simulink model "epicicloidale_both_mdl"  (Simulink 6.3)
settings: Solver=ode45  StartTime=0.0  StopTime=10.0  RelTol=1e-3
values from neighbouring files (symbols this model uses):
  b_c = kb*J_c    (= 4.94590955184)    [architetture_epicicloidale.m]    (also in architetture_epicicloidale_cont.m; architetture_epicicloidale_HEV.m = 92.8974810391; architetture_epicicloidale_prova.m; architetture_HEV_controllo.m = 9.28974810391)
  b_r = kb*J_r    (= 218.026030555)    [architetture_epicicloidale.m]    (also in architetture_epicicloidale_cont.m; architetture_epicicloidale_HEV.m; architetture_epicicloidale_prova.m; architetture_HEV_controllo.m = 21.8026030555)
  b_s = kb*J_s    (= 8.12277148259)    [architetture_epicicloidale.m]    (also in architetture_epicicloidale_cont.m; architetture_epicicloidale_HEV.m = 4.94590955184; architetture_epicicloidale_prova.m; architetture_HEV_controllo.m = 0.494590955184)
  b_sc = kb*J_sc    (= 92.8974810391)    [architetture_epicicloidale.m]    (also in architetture_epicicloidale_cont.m; architetture_epicicloidale_prova.m; epicicloidale.m; epicicloidale_da_solo.m)
  d_cs = d0    (= 10)    [architetture_epicicloidale.m]    (also in architetture_epicicloidale_cont.m; architetture_epicicloidale_prova.m; epicicloidale.m; epicicloidale_da_solo.m)
  d_sr = d0    (= 10)    [architetture_epicicloidale.m]    (also in architetture_epicicloidale_cont.m; architetture_epicicloidale_prova.m; epicicloidale.m; epicicloidale_da_solo.m)
  J_c = 1.3*0.5*pi*rho_acc*hc*r_c^4    (= 0.0494590955184)    [architetture_epicicloidale.m]    (also in architetture_epicicloidale_cont.m; architetture_epicicloidale_HEV.m = 0.928974810391; architetture_epicicloidale_prova.m; architetture_HEV_controllo.m = 0.928974810391)
  J_r = 0.5*pi*rho_acc*(hr*r_ri^4 + h_ring*(r_re^4-r_ri^4))    (= 2.18026030555)    [architetture_epicicloidale.m]    (also in architetture_epicicloidale_cont.m; architetture_epicicloidale_HEV.m; architetture_epicicloidale_prova.m; architetture_HEV_controllo.m)
  J_s = Nr_sat*0.5*pi*rho_acc*(hs*r_s^4 + hc*r_s^4)    (= 0.0812277148259)    [architetture_epicicloidale.m]    (also in architetture_epicicloidale_cont.m; architetture_epicicloidale_HEV.m = 0.0494590955184; architetture_epicicloidale_prova.m; architetture_HEV_controllo.m = 0.0494590955184)
  J_sc = Nr_sat*(r_c+r_s)^2*rho_acc*pi*(hs*r_s^2 + hc*r_s^2)    (= 0.928974810391)    [architetture_epicicloidale.m]    (also in architetture_epicicloidale_cont.m; architetture_epicicloidale_prova.m; epicicloidale.m; epicicloidale_da_solo.m)
  K_cs = K0    (= 10000000)    [architetture_epicicloidale.m]    (also in architetture_epicicloidale_cont.m; architetture_epicicloidale_prova.m; epicicloidale.m; epicicloidale_da_solo.m)
  K_sr = K0    (= 10000000)    [architetture_epicicloidale.m]    (also in architetture_epicicloidale_cont.m; architetture_epicicloidale_prova.m; epicicloidale.m; epicicloidale_da_solo.m)
  Nr_sat = 4    [architetture_epicicloidale.m]    (also in architetture_epicicloidale_cont.m; architetture_epicicloidale_HEV.m; architetture_epicicloidale_prova.m; architetture_HEV_controllo.m)
  r_c = r_ri-2*r_s    (= 0.101859163579)    [architetture_epicicloidale.m]    (also in architetture_epicicloidale_cont.m; architetture_epicicloidale_prova.m; epicicloidale.m; epicicloidale_da_solo.m)
  r_ri = xds*Nr/(2*pi)    (= 0.248281711223)    [architetture_epicicloidale.m]    (also in architetture_epicicloidale_cont.m; architetture_epicicloidale_prova.m; epicicloidale.m; epicicloidale_da_solo.m)
  r_s = xds*Ns/(2*pi)    (= 0.0732112738223)    [architetture_epicicloidale.m]    (also in architetture_epicicloidale_cont.m; architetture_epicicloidale_HEV.m = 0.101859163579; architetture_epicicloidale_prova.m; architetture_HEV_controllo.m = 0.101859163579)
  Tau_c = 0*N*metri    (= 0)    [architetture_epicicloidale.m]    (also in architetture_epicicloidale_cont.m; architetture_epicicloidale_prova.m; epicicloidale.m; epicicloidale_confronto_statico_elastico.m = 10)
  Tau_r = 0*N*metri    (= 0)    [architetture_epicicloidale.m]    (also in architetture_epicicloidale_cont.m; architetture_epicicloidale_prova.m; epicicloidale.m; epicicloidale_confronto_statico_elastico.m = 20)
  Tau_sc = 200*N*metri    (= 200)    [architetture_epicicloidale.m]    (also in architetture_epicicloidale_cont.m = 50; architetture_epicicloidale_prova.m = 50; epicicloidale.m = 4; epicicloidale_da_solo.m = 4)
  Tc = 0.05*ms    (= 5e-05)    [architetture_epicicloidale.m]    (also in architetture_epicicloidale_cont.m; architetture_epicicloidale_HEV.m; architetture_epicicloidale_prova.m; architetture_HEV_controllo.m)
  Wc_0 = 0*0.1*rad/secondo    (= 0)    [architetture_epicicloidale.m]    (also in architetture_epicicloidale_cont.m; architetture_epicicloidale_HEV.m; architetture_epicicloidale_prova.m; Confronto_CVT_EMR.m)
  Wr_0 = Sys1.C(3,:)*[Wc_0; Wsc_0]    [architetture_epicicloidale.m]    (also in Confronto_CVT_EMR.m = 0; epicicloidale.m; epicicloidale_confronto_statico_elastico.m = [-r_s/r_r, 1+r_s/r_r]*[Ws_0; Wc_0]; epicicloidale_da_solo.m = [ -1/r_ri*r_c, (r_c+r_ri)/r_ri]*[Wc_0; Wsc_0])
  Wsc_0 = -0*0.2*rad/secondo    (= 0)    [architetture_epicicloidale.m]    (also in architetture_epicicloidale_cont.m; architetture_epicicloidale_HEV.m; architetture_epicicloidale_prova.m; epicicloidale.m = -0.2)

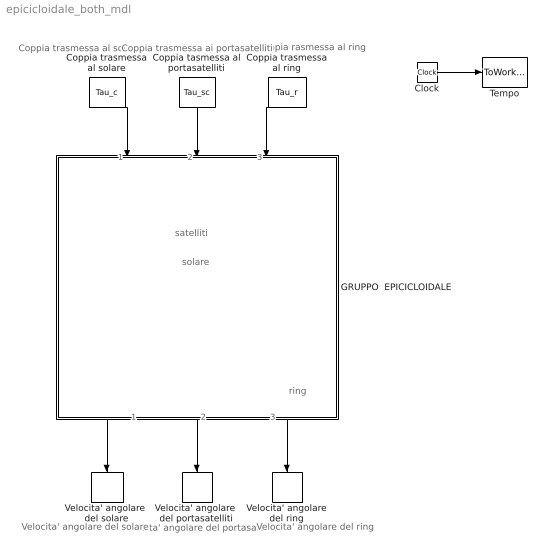
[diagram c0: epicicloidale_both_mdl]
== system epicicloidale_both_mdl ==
  note: solare
  note: satelliti
  note: ring
  note: Velocita' angolare del portasatelliti
  note: Velocita' angolare del ring
  note: Velocita' angolare del solare
  note: Coppia rasmessa al ring
  note: Coppia trasmessa al solare
  note: Coppia trasmessa ai portasatelliti
  Clock : Clock
  Coppia tasmessa al portasatelliti : Constant  Orientation=down  Value=Tau_sc
  Coppia trasmessa al ring : Constant  Orientation=down  Value=Tau_r
  Coppia trasmessa al solare : Constant  Orientation=down  Value=Tau_c
  GRUPPO  EPICICLOIDALE : Subsystem  Orientation=down  mask(POG Gruppo epicicloidale){Par_solare=[J_c, b_c, r_c], Par_satelliti=[J_s, J_sc, b_s, b_sc, r_s, Nr_sat], Par_ring=[J_r, b_r, r_ri], Tipo_di_Modello=Modello ridotto Wc-Wsc, Cond_in_Wc_Wsc=[Wc_0,  Wsc_0], Cond_in_Wsc_Wr=[Wsc_0,  Wr_0], Cond_in_Wc_Wr=[Wc_0,  Wr_0], Solare_Satelliti=[K_cs, d_cs], Satelliti_Ring=[K_sr, d_sr], Cond_in=[Wc_0, Wsc_0,Wr_0]}
      mask prompts: Par_solare "Parametri Solare: [J_c, b_c, r_c]-->[kg*m^2,N*m*s/rad,m]"; Par_satelliti "Parametri Satelliti: [J_s, J_sc, b_s, b_sc, r_s, Nr_sat]-->[kg*m^2,N*m*s/rad,m]"; Par_ring "Parametri Ring: [J_r, b_r, r_ri]-->[kg*m^2,N*m*s/rad,m,m]"; Tipo_di_Modello "Tipo di modello"; Cond_in_Wc_Wsc "Condizioni iniziali: [Wc_0,  Wsc_0]-->[rad/s]"; Cond_in_Wsc_Wr "Condizioni iniziali: [Wsc_0,  Wr_0]-->[rad/s]"; Cond_in_Wc_Wr "Condizioni iniziali: [Wc_0,  Wr_0]-->[rad/s]"; Solare_Satelliti "Solare-Satelliti: [K_cs, d_cs]-->[N/m,N*m*s/rad]"; Satelliti_Ring "Satelliti-Ring: [K_sr, d_sr]-->[N/m,N*m*s/rad]"; Cond_in "Condizioni iniziali: [Wc_0,  Wsc_0, Wr_0]-->[rad/s]"
      mask help: Gruppo epicicloidale: [J_c, J_s, J_r, J_sc]= Inerzie di: solare, satelliti, ring, solare-ssatelliti; [b_c, b_s, b_r]= Attriti di: solare, satelliti, ring; [r_c, r_s, r_ri, r_re]= Raggi di: solare, satelliti, ring(interno ed esterno); [Nr_sat]= Numero Satelliti; [K_cs, K_sr]= Elasticita' tra solare-satelliti e tra satelliti-ring; [b_sc]= Attriti tra solare-satelliti; [d_cs, d_sr]= Elementi della matrice D; [Wc_0, Wsc_0, Wr_0]=Velocita' iniziali di solare, satelliti, portasatelliti, ring;
      mask init:
      | J_c=double(Par_solare(1));          
      | b_c=double(Par_solare(2));            
      | r_c=double(Par_solare(3));           
      | %
      | J_s=double(Par_satelliti(1));            
      | J_sc=double(Par_satelliti(2));            
      | b_s=double(Par_satelliti(3));            
      | b_sc=double(Par_satelliti(4));            
      | r_s=double(Par_satelliti(5));            
      | Nr_sat=double(Par_satelliti(6));           
      | %
      | J_r=double(Par_ring(1));             
      | b_r=double(Par_ring(2));            
      | r_ri=double(Par_ring(3));                  
      | %
      | %%%%%%%%%%%%%%%%%%%%%%%%%%%%%%%%%%%%%%%%%%%%%%%%%%%%%%%%%%%%%%%%%%%%%%%%%%%
      | %   Modello esteso e modelli ridotti
      | %%%%%%%%%%%%%%%%%%%%%%%%%%%%%%%%%%%%%%%%%%%%%%%%%%%%%%%%%%%%%%%%%%%%%%%%%%%
      | if Tipo_di_Modello=='Modello esteso        '
      |     %
      |     K_cs=double(Solare_Satelliti(1));
      |     d_cs=double(Solare_Satelliti(2));
      |     if(K_cs==0)
      |         K_cs=inf;
      |     end
      |     %
      |     K_sr=double(Satelliti_Ring(1));
      |     d_sr=double(Satelliti_Ring(2));
      |     if(K_sr==0)
      |         K_sr=inf;
      |     end
      |     %
      |     %
      |     L=[ J_c,      0,      0,      0,      0,      0;
      |           0, 1/K_cs,      0,      0,      0,      0;
      |           0,      0,    J_s,      0,      0,      0;
      |           0,      0,      0,   J_sc,      0,      0;
      |           0,      0,      0,      0, 1/K_sr,      0;
      |           0,      0,      0,      0,      0,    J_r];
      |     %
      |     A=- [-b_c-r_c^2*d_cs,    -r_c,                -r_c*d_cs*r_s,                   r_c^2*d_cs,      0,                  0;
      |         r_c,                    0,                          r_s,                         -r_c,      0,                  0;
      |         -r_c*d_cs*r_s,       -r_s,   -b_s-d_cs*r_s^2-d_sr*r_s^2,   r_c*d_cs*r_s-d_sr*r_s*r_ri,   -r_s,      d_sr*r_s*r_ri;
      |         r_c^2*d_cs,           r_c,   r_c*d_cs*r_s-d_sr*r_s*r_ri, -b_sc-r_c^2*d_cs-d_sr*r_ri^2,  -r_ri,        d_sr*r_ri^2;
      |         0,                      0,                          r_s,                         r_ri,      0,              -r_ri;
      |         0,                      0,                d_sr*r_s*r_ri,                  d_sr*r_ri^2,   r_ri,   -b_r-d_sr*r_ri^2];
      |     %
      |     B=[ 1, 0, 0;
      |         0, 0, 0;
      |         0, 0, 0;
      |         0, 1, 0;
      |         0, 0, 0;
      |         0, 0, 1];
      |     %
      |     C=[ 1, 0, 0, 0, 0, 0;
      |         0, 0, 0, 1, 0, 0;
      |         0, 0, 0, 0, 0, 1];
      |     %
      |     Wc_0=double(Cond_in(1));
      |     Wsc_0=double(Cond_in(2));
      |     Wr_0=double(Cond_in(3));
      |     Ws_0=r_c*(Wsc_0-Wc_0)/r_s;
      |     Ws_sc_0=[Ws_0 Wsc_0];
      |     %
      |     We_0=[Wc_0 0 Ws_sc_0 0 Wr_0 ];
      |     %
      | elseif Tipo_di_Modello=='Modello ridotto Wc-Wsc'
      |     L = [ (J_c*r_s^2*r_ri^2+r_ri^2*r_c^2*J_s+J_r*r_s^2*r_c^2)/r_s^2/r_ri^2,                                        -r_c*(r_ri^2*r_c*J_s+J_r*r_s^2*r_c+J_r*r_s^2*r_ri)/r_s^2/r_ri^2;
      |           -r_c*(r_ri^2*r_c*J_s+J_r*r_s^2*r_c+J_r*r_s^2*r_ri)/r_s^2/r_ri^2, (J_r*r_s^2*r_c^2+2*J_r*r_s^2*r_ri*r_c+J_r*r_s^2*r_ri^2+r_ri^2*r_c^2*J_s+r_ri^2*J_sc*r_s^2)/r_s^2/r_ri^2];
      |     %
      |     A=-[ -(b_c*r_s^2*r_ri^2+r_c^2*r_ri^2*b_s+b_r*r_s^2*r_c^2)/r_s^2/r_ri^2,                                          r_c*(r_c*r_ri^2*b_s+b_r*r_s^2*r_c+b_r*r_s^2*r_ri)/r_s^2/r_ri^2;
      |         r_c*(r_c*r_ri^2*b_s+b_r*r_s^2*r_c+b_r*r_s^2*r_ri)/r_s^2/r_ri^2,    -(b_sc*r_s^2*r_ri^2+r_c^2*r_ri^2*b_s+b_r*r_s^2*r_c^2+2*b_r*r_s^2*r_c*r_ri+b_r*r_s^2*r_ri^2)/r_s^2/r_ri^2];
      |     %
      |     B= [  1,    0,     -1/r_ri*r_c;
      |           0,    1, (r_c+r_ri)/r_ri];
      |     %
      |     C= [            1,               0;
      |                     0,               1;
      |           -1/r_ri*r_c, (r_c+r_ri)/r_ri];
      |     %
      |     Wc_0=double(Cond_in_Wc_Wsc(1));
      |     Wsc_0=double(Cond_in_Wc_Wsc(2));
      |     We_0=[Wc_0 Wsc_0];
      |     %
      | elseif Tipo_di_Modello=='Modello ridotto Wsc-Wr'
      |     L= [ (J_sc*r_c^2*r_s^2+J_c*r_s^2*r_c^2+2*J_c*r_s^2*r_c*r_ri+J_c*r_s^2*r_ri^2+r_ri^2*J_s*r_c^2)/r_c^2/r_s^2,   -r_ri*(J_c*r_s^2*r_c+J_c*r_s^2*r_ri+r_ri*J_s*r_c^2)/r_c^2/r_s^2;
      |          -r_ri*(J_c*r_s^2*r_c+J_c*r_s^2*r_ri+r_ri*J_s*r_c^2)/r_c^2/r_s^2,                                        (J_r*r_c^2*r_s^2+J_c*r_s^2*r_ri^2+r_ri^2*J_s*r_c^2)/r_c^2/r_s^2];
      | 
      |     A=-[ -(b_sc*r_c^2*r_s^2+b_c*r_s^2*r_c^2+2*b_c*r_s^2*r_c*r_ri+b_c*r_s^2*r_ri^2+r_ri^2*b_s*r_c^2)/r_c^2/r_s^2,     r_ri*(b_c*r_s^2*r_c+b_c*r_s^2*r_ri+r_ri*b_s*r_c^2)/r_c^2/r_s^2;
      |          r_ri*(b_c*r_s^2*r_c+b_c*r_s^2*r_ri+r_ri*b_s*r_c^2)/r_c^2/r_s^2,                                          -(b_r*r_c^2*r_s^2+b_c*r_s^2*r_ri^2+r_ri^2*b_s*r_c^2)/r_c^2/r_s^2];
      | 
      |     B= [ (r_c+r_ri)/r_c,    1,   0;
      |             -1/r_c*r_ri,    0,   1];
      | 
      |     C= [ (r_c+r_ri)/r_c,  -1/r_c*r_ri;
      |                       1,            0;
      |                       0,            1];
      |     %
      |     Wsc_0=double(Cond_in_Wsc_Wr(1));
      |     Wr_0=double(Cond_in_Wsc_Wr(2));
      |     We_0=[Wsc_0 Wr_0];
      |     %
      | elseif Tipo_di_Modello=='Modello ridotto  Wc-Wr'
      |     L= [ (J_c*r_s^2*r_c^2+2*J_c*r_s^2*r_c*r_ri+J_c*r_s^2*r_ri^2+r_ri^2*r_c^2*J_s+r_c^2*J_sc*r_s^2)/r_s^2/(r_c+r_ri)^2,                                                        r_c*r_ri*(-r_ri*r_c*J_s+J_sc*r_s^2)/r_s^2/(r_c+r_ri)^2;
      |           r_c*r_ri*(-r_ri*r_c*J_s+J_sc*r_s^2)/r_s^2/(r_c+r_ri)^2,                                                      (J_r*r_s^2*r_c^2+2*J_r*r_s^2*r_c*r_ri+J_r*r_s^2*r_ri^2+r_ri^2*r_c^2*J_s+r_ri^2*J_sc*r_s^2)/r_s^2/(r_c+r_ri)^2];
      | 
      |     A=-[-(b_c*r_s^2*r_c^2+2*b_c*r_s^2*r_c*r_ri+b_c*r_s^2*r_ri^2+r_c^2*r_ri^2*b_s+r_c^2*r_s^2*b_sc)/r_s^2/(r_c+r_ri)^2,                                                        -r_c*r_ri*(-r_c*r_ri*b_s+r_s^2*b_sc)/r_s^2/(r_c+r_ri)^2;
      |         -r_c*r_ri*(-r_c*r_ri*b_s+r_s^2*b_sc)/r_s^2/(r_c+r_ri)^2,                                                       -(b_r*r_s^2*r_c^2+2*b_r*r_s^2*r_c*r_ri+b_r*r_s^2*r_ri^2+r_c^2*r_ri^2*b_s+r_ri^2*r_s^2*b_sc)/r_s^2/(r_c+r_ri)^2];
      | 
      |     B=[   1,  1/(r_c+r_ri)*r_c, 0;
      |           0, 1/(r_c+r_ri)*r_ri, 1];
      | 
      |     C=[                 1,                  0;
      |          1/(r_c+r_ri)*r_c,  1/(r_c+r_ri)*r_ri;
      |                         0,                  1];
      |     Wc_0=double(Cond_in_Wc_Wr(1));
      |     Wr_0=double(Cond_in_Wc_Wr(2));
      |     We_0=[Wc_0 Wr_0];
      | end
  Tempo : ToWorkspace  VariableName=t  SampleTime=Tc  SaveFormat=Array
  Velocita' angolare del ring : ToWorkspace  VariableName=W_r  SampleTime=Tc  SaveFormat=Array
  Velocita' angolare  del portasatelliti : ToWorkspace  VariableName=W_sc  SampleTime=Tc  SaveFormat=Array
  Velocita' angolare  del solare : ToWorkspace  VariableName=W_c  SampleTime=Tc  SaveFormat=Array
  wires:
  Clock/1 -> Tempo/1
  Coppia trasmessa al solare/1 -> GRUPPO  EPICICLOIDALE/1(Tau_c)
  Coppia tasmessa al portasatelliti/1 -> GRUPPO  EPICICLOIDALE/2(Tau_sc)
  Coppia trasmessa al ring/1 -> GRUPPO  EPICICLOIDALE/3(Tau_r)
  GRUPPO  EPICICLOIDALE/3(w_r) -> Velocita' angolare del ring/1
  GRUPPO  EPICICLOIDALE/2(w_sc) -> Velocita' angolare  del portasatelliti/1
  GRUPPO  EPICICLOIDALE/1(w_c) -> Velocita' angolare  del solare/1

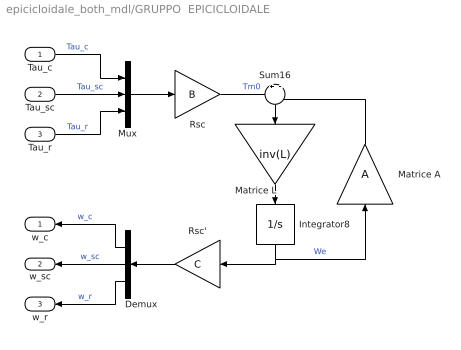
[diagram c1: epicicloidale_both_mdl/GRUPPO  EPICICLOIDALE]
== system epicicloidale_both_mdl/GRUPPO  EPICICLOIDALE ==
  Tau_c : Inport
  Tau_sc : Inport  Port=2
  Tau_r : Inport  Port=3
  Demux : Demux  Orientation=left  Outputs=3
  Integrator8 : Integrator  Orientation=down  InitialCondition=We_0  LowerSaturationLimit=0
  Matrice A : Gain  Orientation=up  Gain=A  Multiplication=Matrix(K*u)
  Matrice L : Gain  Orientation=down  Gain=inv(L)  Multiplication=Matrix(K*u)
  Mux : Mux  Inputs=3
  Rsc : Gain  Gain=B  Multiplication=Matrix(K*u)
  Rsc' : Gain  Orientation=left  Gain=C  Multiplication=Matrix(K*u)
  Sum16 : Sum  Orientation=down  Inputs=+|-
  w_c : Outport  Orientation=left
  w_sc : Outport  Orientation=left  Port=2
  w_r : Outport  Orientation=left  Port=3
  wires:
  Rsc/1 -> Sum16/1  "Tm0"
  Sum16/1 -> Matrice L/1
  Matrice L/1 -> Integrator8/1
  Integrator8/1 -> Matrice A/1, Rsc'/1  "We"
  Matrice A/1 -> Sum16/2
  Tau_c/1 -> Mux/1  "Tau_c"
  Tau_sc/1 -> Mux/2  "Tau_sc"
  Tau_r/1 -> Mux/3  "Tau_r"
  Mux/1 -> Rsc/1
  Rsc'/1 -> Demux/1
  Demux/1 -> w_c/1  "w_c"
  Demux/2 -> w_sc/1  "w_sc"
  Demux/3 -> w_r/1  "w_r"
